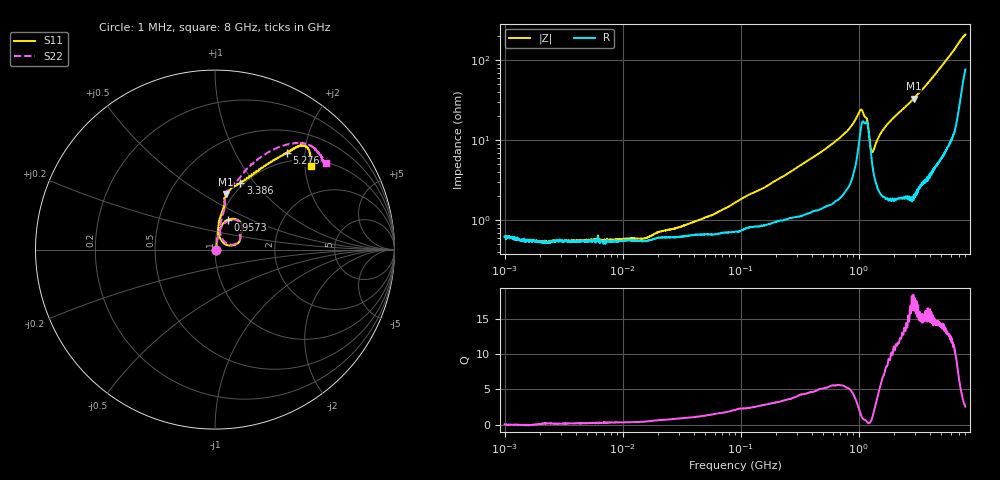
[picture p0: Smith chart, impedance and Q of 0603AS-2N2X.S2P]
!s-Parameter Generated by FASTRON Sdn. Bhd.
!FASTRON P/N : 0603AS-2N2X
!Keysight Technologies: E5071C_MY46733604_B.14.02
!Date: Tue Oct 24 10:22:04 2023
!Version  :Rev01  Tue Oct 24 10:22:04 2023
!Data & Calibration Information:
!Freq  S11:SOLT2(ON)  S21:SOLT2(ON)  S12:SOLT2(ON)  S22:SOLT2(ON)
!PortZ  Port1:50+j0  Port2:50+j0
!When reading reference impedance value at option line is always used.
! Remarks : This data is being provided solely for informational purposes.
# Hz S dB R 50
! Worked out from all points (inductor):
!   1601 points, 1 MHz to 8 GHz, reference 50 ohm
!   read as one part in series: L = 2.36 nH near 181.9 MHz
!   highest Q = 16.9 at 2.912 GHz (marker M1), where L = 1.8 nH
!   S11 on the Smith chart (normalised r, x): 1 MHz: 1.01, -0.00; 957.3 MHz: 1.09, +0.37; 3.386 GHz: 0.96, +0.85; 5.276 GHz: 0.85, +1.66; 8 GHz: 1.16, +2.14
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1000000  -43.54 -3.6  -0.05 -0.1  -0.05 0.0  -43.76 1.2
1541011  -46.56 -10.4  -0.05 -0.1  -0.05 -0.0  -44.08 -18.4
2286470  -45.05 10.6  -0.05 -0.0  -0.05 -0.1  -47.82 12.1
2905262  -45.92 5.3  -0.06 -0.1  -0.05 -0.0  -46.51 4.1
4479405  -45.44 9.8  -0.05 -0.1  -0.05 -0.1  -46.65 12.1
8407329  -45.06 14.2  -0.05 -0.1  -0.05 -0.1  -45.46 14.7
1.518223e7  -49.98 -1.4  -0.04 -0.2  -0.06 -0.2  -43.08 17.0
2.00676e7  -43.79 30.0  -0.05 -0.3  -0.06 -0.2  -42.94 36.6
6.021717e7  -39.04 58.1  -0.06 -0.6  -0.06 -0.6  -38.76 54.4
8.994653e7  -35.86 65.5  -0.06 -0.9  -0.07 -0.9  -36.21 62.6
4.006501e8  -24.47 77.4  -0.14 -3.2  -0.15 -3.3  -24.46 76.3
9.573479e8  -14.87 66.8  -0.68 -9.6  -0.68 -9.6  -14.89 64.5
1.035959e9  -13.60 49.7  -1.29 -9.6  -1.30 -9.7  -13.72 47.7
1.1258e9  -15.58 31.1  -1.42 -5.0  -1.43 -5.1  -15.77 32.6
1.303145e9  -24.02 55.7  -0.50 -2.4  -0.51 -2.5  -23.16 49.7
1.511962e9  -18.59 81.2  -0.35 -6.1  -0.35 -6.2  -18.58 76.7
1.7949e9  -15.74 82.0  -0.40 -8.9  -0.40 -9.0  -15.78 78.2
2.912392e9  -10.03 79.3  -1.20 -17.0  -1.21 -17.0  -10.03 79.4
3.385893e9  -7.98 69.3  -1.34 -19.5  -1.34 -19.6  -7.99 72.8
5.276366e9  -3.49 53.3  -3.79 -32.3  -3.78 -32.4  -3.35 57.6
6.766244e9  -2.35 49.2  -6.88 -37.9  -6.87 -38.2  -2.05 47.3
8e9  -3.02 41.1  -9.76 -32.9  -9.75 -33.3  -2.12 38.0
